(* SV dataset values buffer type (IEC 61850 big endian network byte order) *)
{attribute 'pack_mode' := '1'}
TYPE ST_SVDATA_IED_MUnn_LLN0_PhsMeas1 : 
STRUCT
	IED_MUnn_InnATCTR1_AmpSv_instMag_i: T_OCTET4;
	IED_MUnn_InnATCTR1_AmpSv_q: T_OCTET4;
	IED_MUnn_InnBTCTR2_AmpSv_instMag_i: T_OCTET4;
	IED_MUnn_InnBTCTR2_AmpSv_q: T_OCTET4;
	IED_MUnn_InnCTCTR3_AmpSv_instMag_i: T_OCTET4;
	IED_MUnn_InnCTCTR3_AmpSv_q: T_OCTET4;
	IED_MUnn_InnNTCTR4_AmpSv_instMag_i: T_OCTET4;
	IED_MUnn_InnNTCTR4_AmpSv_q: T_OCTET4;
	IED_MUnn_UnnATVTR1_VolSv_instMag_i: T_OCTET4;
	IED_MUnn_UnnATVTR1_VolSv_q: T_OCTET4;
	IED_MUnn_UnnBTVTR2_VolSv_instMag_i: T_OCTET4;
	IED_MUnn_UnnBTVTR2_VolSv_q: T_OCTET4;
	IED_MUnn_UnnCTVTR3_VolSv_instMag_i: T_OCTET4;
	IED_MUnn_UnnCTVTR3_VolSv_q: T_OCTET4;
	IED_MUnn_UnnNTVTR4_VolSv_instMag_i: T_OCTET4;
	IED_MUnn_UnnNTVTR4_VolSv_q: T_OCTET4;
END_STRUCT
END_TYPE
